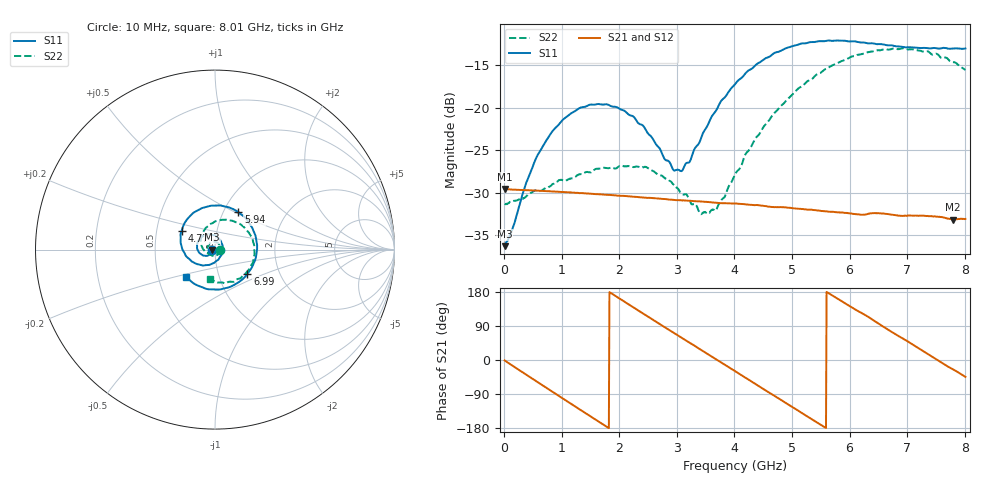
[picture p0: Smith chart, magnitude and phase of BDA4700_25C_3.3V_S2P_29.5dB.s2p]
!Agilent Technologies,E5071B,MY42404982,A.09.10
!Date: Mon Oct 20 18:15:28 2025
!Data & Calibration Information:
!Freq	S11:SOLT2(ON)	S21:SOLT2(ON)	S12:SOLT2(ON)	S22:SOLT2(ON)
# Hz S RI R 50
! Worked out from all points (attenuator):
!   801 points, 10 MHz to 8.01 GHz, reference 50 ohm
!   highest |S21| = -29.55 dB at 20 MHz (marker M1); lowest = -33.1 dB at 7.79 GHz (marker M2)
!   lowest |S11| = -36.3 dB at 10 MHz (marker M3), VSWR 1.03, Z = 48.5 - j0.116 ohm
!   |S11| at or under -10 dB: start of sweep to end of sweep
!   |S22| runs from -32.5 to -13.0 dB; largest |S21 - S12| = 0.00042
!   S11 on the Smith chart (normalised r, x): 10 MHz: 0.97, -0.00; 4.77 GHz: 0.67, +0.15; 5.94 GHz: 1.17, +0.52; 6.99 GHz: 1.38, -0.39; 8.01 GHz: 0.69, -0.22
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1e7  -0.0153 -0.00119  0.0333 -0.000732  0.0333 -0.000762  0.0272 -0.000827
2e7  -0.0157 -0.00193  0.0333 -0.00124  0.0332 -0.0014  0.0271 -0.0011
5.9e8  -0.0408 -0.0342  0.0168 -0.0279  0.0168 -0.0279  0.0139 -0.0295
1.01e9  -0.0807 -0.0243  -0.00584 -0.0314  -0.00583 -0.0314  -0.0151 -0.0345
1.35e9  -0.1001 0.00902  -0.0218 -0.0227  -0.0218 -0.0227  -0.0364 -0.0183
2.07e9  -0.049 0.083  -0.0277 0.0124  -0.0277 0.0124  -0.031 0.0332
2.68e9  0.0318 0.0495  -0.00359 0.0291  -0.0037 0.0291  0.0127 0.0384
2.94e9  0.0422 0.00889  0.00872 0.0274  0.00873 0.0273  0.0253 0.0249
3.09e9  0.039 -0.0171  0.0152 0.0242  0.015 0.0243  0.0284 0.0129
3.41e9  0.00612 -0.0643  0.0249 0.0132  0.025 0.0131  0.0213 -0.0108
3.55e9  -0.0176 -0.0787  0.0271 0.00692  0.0271 0.00685  0.0132 -0.02
3.7e9  -0.0482 -0.0859  0.0276 0.000101  0.0277 3.82e-06  0.000482 -0.0258
4.01e9  -0.116 -0.0729  0.0239 -0.0134  0.0239 -0.0133  -0.031 -0.0259
4.77e9  -0.1862 0.1028  -0.00529 -0.0255  -0.00516 -0.0256  -0.0779 0.0609
5.35e9  -0.0657 0.2333  -0.0231 -0.00989  -0.023 -0.01  -0.016 0.1466
5.94e9  0.1305 0.2087  -0.0204 0.0129  -0.0205 0.0127  0.1159 0.1526
6.37e9  0.2225 0.086  -0.00786 0.0226  -0.00794 0.0225  0.1967 0.0803
6.68e9  0.2302 -0.0294  0.00456 0.0233  0.00461 0.0232  0.219 0.000544
6.99e9  0.181 -0.1349  0.0147 0.0179  0.0148 0.018  0.2047 -0.082
7.43e9  0.0389 -0.2196  0.0227 0.00363  0.0228 0.00358  0.12 -0.1662
7.79e9  -0.0967 -0.2001  0.0201 -0.00905  0.0201 -0.00916  0.0231 -0.1833
8.01e9  -0.1626 -0.1514  0.0158 -0.0156  0.0159 -0.0156  -0.0293 -0.1634
